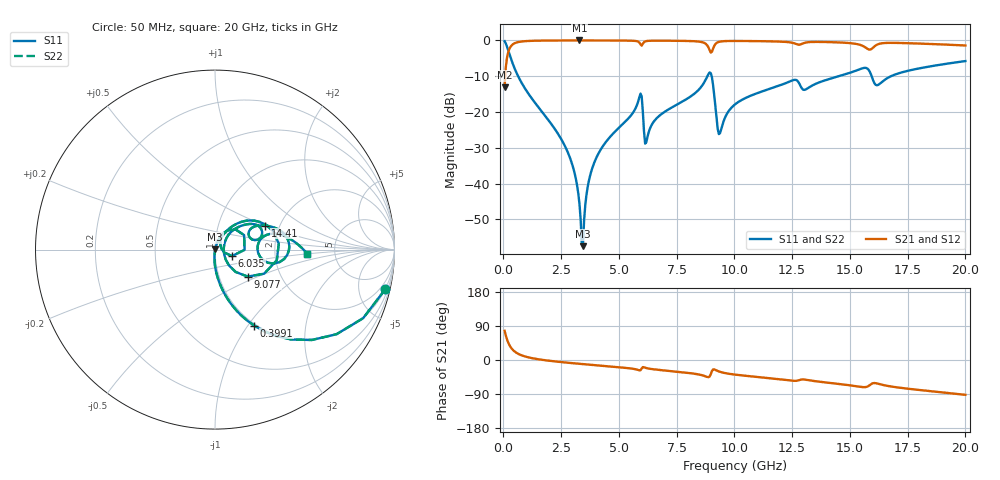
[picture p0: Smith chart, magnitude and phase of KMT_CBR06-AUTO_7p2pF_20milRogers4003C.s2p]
! Data measured by Modelithics Inc. support@modelithics.com 813-866-6335
! KEMET CBR06-AUTO 7.2pF, Pad Width= 0.851mm, Pad Length= 0.64mm, Pad Gap= 0.62mm, 20mil Rogers 4003C substrate Data, January 2022
# hz S ma R 50
! 2 Port Network Data from SP1.SP block
! freq  magS11  angS11  magS21  angS21  magS12  angS12  magS22  angS22
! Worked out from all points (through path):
!   401 points, 50 MHz to 20 GHz, reference 50 ohm
!   highest |S21| = -0.01 dB at 3.292 GHz (marker M1); lowest = -13.1 dB at 50 MHz (marker M2)
!   group delay of S21, straight-line fit = 14.1 ps
!   lowest |S11| = -57.5 dB at 3.442 GHz (marker M3), VSWR 1.00, Z = 50.1 + j0.075 ohm
!   |S11| at or under -10 dB: 635.8 MHz to 8.828 GHz (8.192 GHz wide, 173 % of centre); 9.014 GHz to 14.52 GHz (5.502 GHz wide, 46.8 % of centre); 15.94 GHz to 16.78 GHz (836.6 MHz wide, 5.11 % of centre)
!   |S22| runs from -57.5 to -0.2 dB; largest |S21 - S12| = 0
!   S11 on the Smith chart (normalised r, x): 50 MHz: 0.98, -8.66; 399.1 MHz: 0.98, -1.07; 6.035 GHz: 1.21, -0.09; 9.077 GHz: 1.37, -0.44; 14.41 GHz: 1.68, +0.50; 20 GHz: 3.11, -0.20
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5e7  0.9749 -13.0  0.2225 77.0  0.2225 77.0  0.9749 -13.0
3.99125e8  0.4763 -62.7  0.8787 27.2  0.8787 27.2  0.4763 -62.7
2.74325e9  0.02949 -95.3  0.9986 -6.9  0.9986 -6.9  0.02949 -95.3
3.092375e9  0.01352 -95.1  0.9989 -9.0  0.9989 -9.0  0.01352 -95.1
3.291875e9  0.005176 -89.7  0.9989 -10.1  0.9989 -10.1  0.005176 -89.7
3.391625e9  0.001409 -58.5  0.9989 -10.6  0.9989 -10.6  0.001409 -58.5
3.4415e9  0.001341 33.9  0.9989 -10.9  0.9989 -10.9  0.001341 33.9
3.74075e9  0.01256 72.9  0.9988 -12.5  0.9988 -12.5  0.01256 72.9
4.13975e9  0.02735 73.1  0.9984 -14.6  0.9984 -14.6  0.02735 73.1
5.885375e9  0.1614 43.0  0.9335 -27.2  0.9335 -27.2  0.1614 43.0
6.035e9  0.1017 -20.7  0.8982 -18.7  0.8982 -18.7  0.1017 -20.7
6.184625e9  0.03784 36.2  0.9789 -21.2  0.9789 -21.2  0.03784 36.2
6.73325e9  0.08785 61.5  0.9922 -26.1  0.9922 -26.1  0.08785 61.5
8.678375e9  0.2551 39.5  0.9284 -41.7  0.9284 -41.7  0.2551 39.5
9.077375e9  0.2365 -39.5  0.7691 -24.9  0.7691 -24.9  0.2365 -39.5
9.376625e9  0.05078 13.7  0.9631 -31.3  0.9631 -31.3  0.05078 13.7
1.0025e10  0.1278 47.8  0.9833 -38.5  0.9833 -38.5  0.1278 47.8
1.336662e10  0.2345 30.4  0.9523 -54.8  0.9523 -54.8  0.2345 30.4
1.4414e10  0.3093 25.7  0.9404 -62.4  0.9404 -62.4  0.3093 25.7
1.591025e10  0.3359 -13.4  0.7517 -63.9  0.7517 -63.9  0.3359 -13.4
1.670825e10  0.3086 16.0  0.9248 -69.1  0.9248 -69.1  0.3086 16.0
2e10  0.5153 -2.7  0.8496 -91.9  0.8496 -91.9  0.5153 -2.7
